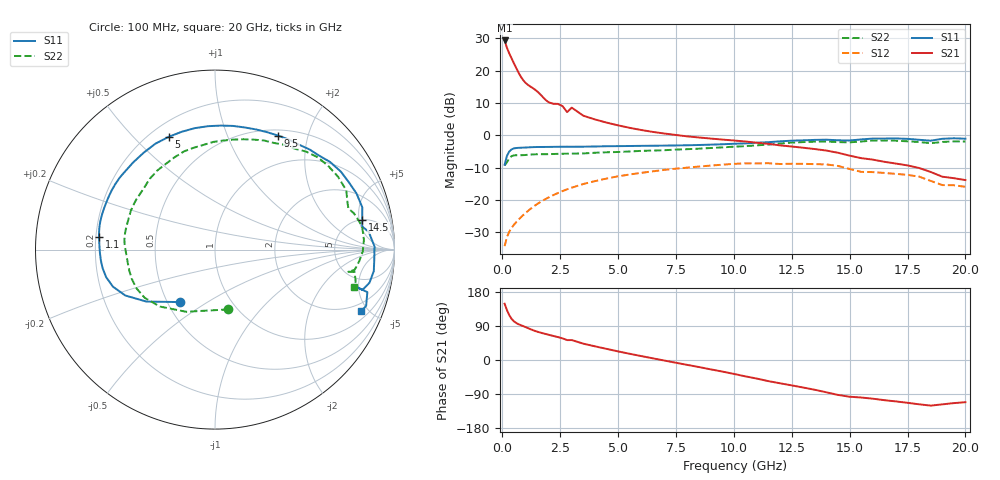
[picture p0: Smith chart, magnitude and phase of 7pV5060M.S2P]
! Infineon Technologies  Discrete & RF Semiconductors
! bfp620
! VCE = 0.50 V,  IC =  60 mA
! Common Emitter S-Parameters:  Sep 2002
# GHz  S  MA  R  50
!  f  S11  S21  S12  S22
! GHz  MAG  ANG  MAG  ANG  MAG  ANG  MAG  ANG
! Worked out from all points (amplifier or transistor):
!   59 points, 100 MHz to 20 GHz, reference 50 ohm
!   highest |S21| = 29.3 dB at 100 MHz (marker M1)
!   |S21| within 3 dB of that: start of sweep to 242.4 MHz
!   unconditionally stable (mu >= 1): 1.485 GHz to 11.42 GHz; 16.33 GHz to end of sweep
!   at 1 GHz: K = 0.99, MSG = 20.1 dB, |S12| = -24.1 dB
!   at 5.5 GHz: K = 1.11, MAG = 5.2 dB, |S12| = -12.1 dB
!   at 20 GHz: K = 1.91, MAG = -4.5 dB, |S12| = -15.9 dB
!   S11 on the Smith chart (normalised r, x): 100 MHz: 0.58, -0.39; 1.1 GHz: 0.21, +0.05; 5 GHz: 0.27, +0.64; 9.5 GHz: 0.57, +1.54; 14.5 GHz: 5.03, +5.55; 20 GHz: 1.43, -4.51
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0.1  0.3502 -123.4  29.21 148.5  0.0193 37.0  0.3415 -77.5
0.2  0.48 -142.9  22.5 131.8  0.0266 39.2  0.3821 -115.0
0.3  0.5613 -152.9  18.44 118.3  0.0323 41.3  0.4413 -134.0
0.4  0.6048 -160.0  15.47 108.7  0.037 43.3  0.4748 -145.5
0.5  0.6257 -165.8  13.02 102.1  0.0412 45.2  0.4883 -154.0
0.6  0.6349 -170.7  10.97 97.7  0.0453 46.9  0.4916 -160.8
0.8  0.6414 -178.4  8.043 91.9  0.0537 49.4  0.4916 -170.9
1.1  0.6497 173.9  6.037 84.4  0.0673 51.3  0.4989 -179.9
1.5  0.6581 165.9  4.789 74.9  0.0861 51.1  0.5089 171.6
2  0.6603 156.2  3.238 66.6  0.1094 48.5  0.5106 161.2
2.6  0.6645 147.0  2.825 57.2  0.1371 43.7  0.518 152.2
2.8  0.6652 143.3  2.281 52.5  0.1459 41.9  0.5194 148.2
3  0.6645 141.0  2.673 52.6  0.155 39.9  0.5199 146.7
3.5  0.6662 133.2  2.005 43.1  0.1763 34.7  0.5234 139.2
5  0.6792 112.3  1.423 22.7  0.2323 19.0  0.5512 119.3
7  0.6919 87.2  1.064 -1.4  0.2917 -1.9  0.5874 96.0
9.5  0.726 61.0  0.858 -30.5  0.3509 -29.0  0.6492 70.7
10.5  0.749 51.3  0.801 -43.2  0.3681 -41.6  0.6785 61.2
13.5  0.8483 21.6  0.612 -78.6  0.3578 -76.1  0.7969 30.6
14.5  0.8368 11.4  0.536 -92.2  0.3355 -91.4  0.7839 19.7
17  0.8928 -7.7  0.365 -109.3  0.2529 -106.8  0.8232 -0.8
20  0.8844 -22.9  0.203 -111.3  0.1597 -118.5  0.8013 -15.0
